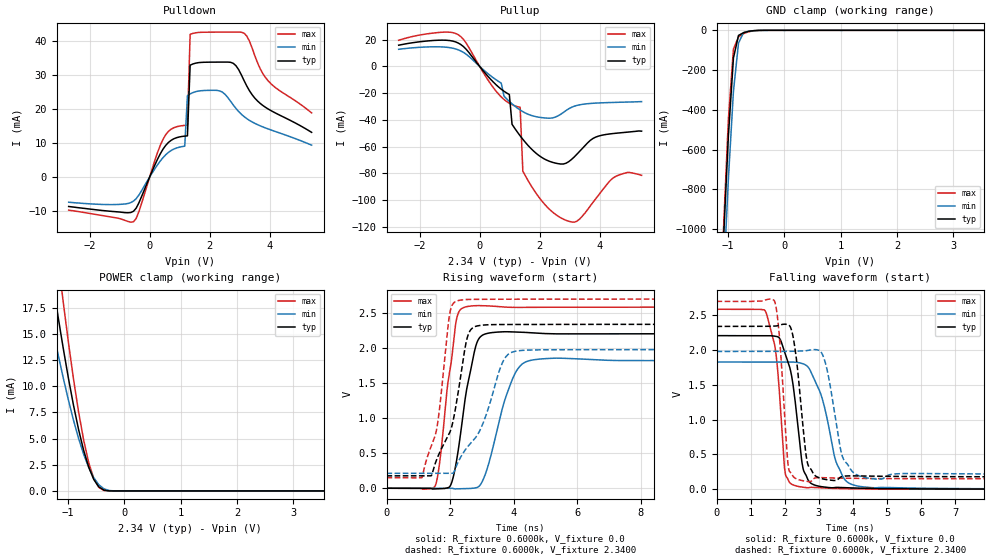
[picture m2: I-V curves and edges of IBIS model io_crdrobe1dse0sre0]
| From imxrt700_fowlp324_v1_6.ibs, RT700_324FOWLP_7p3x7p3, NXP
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[Model] io_crdrobe1dse0sre0
|   Model io_crdrobe1dse0sre0
| This model was characterised for following simulation conditions:
| External (pad) voltage:
|   - Typ: 2.34V,   - Min: 1.98V,   - Max: 2.7V
| Library cells for typ/min/max conditions are connected as defined below:
|  PAD_IO - External Pad
|  ipp_do - Core Input
|  ipp_obe - Output Buffer Enable
|  ASRCN3V3[3] - NC
|  ASRCN3V3[4] - NC
|  ASRCP3V3[4] - NC
|  REFAPBIAS3V3 - gnde
|  REFBAMPL3V3 - vdd1v8
|  REFCAMPH3V3 - vdd1v8
|  REFDNBIAS3V3 - vdd1v8
|  REFH3V3 - REFH3V3
|  REFL3V3 - REFL3V3
|  gnde - gnde
|  ipp_dse - gnde
|  ipp_ina235_3v - NC
|  ipp_ina40_3v - NC
|  ipp_ina_mux - NC
|  ipp_ind - NC
|  ipp_ind_1p8v - NC
|  ipp_ind_3v - NC
|  ipp_sre - gnde
|  vdd - vdd
|  vdd1v8 - vdd1v8
|  vdda - vdde3v3
|  vdde3v3 - vdde3v3
| All other pins connected to ground
Model_type I/O
Polarity   Non-Inverting
Enable   Active-High
Vinl =   0.7020V
Vinh =   1.6300V
Vmeas =  1.1700V
Cref =   15.0000pF
Rref =   0.6000k
Vref =   0.0V
C_comp   3.9951pF   3.8194pF   4.1033pF
|C_comp_pullup   0.5141pF   0.5880pF   0.4995pF
|C_comp_pulldown   2.0718pF   2.1610pF   1.8544pF
[Model Spec]
| variable   typ   min   max
Vinh   1.6300V   NA   NA
Vinl   0.7020V   NA   NA
Vref   0.0V   0.0V   0.0V
Cref   15.0000pF   15.0000pF   15.0000pF
Rref   0.6000k   0.6000k   0.6000k
[Receiver Thresholds]
Vcross_high  =   0.0V
Vcross_low  =   0.0V
Vdiff_ac  =   0.0V
Vdiff_dc  =   0.0V
Tdiffslew_ac  =   0.0S
[Temperature Range]   25.0000   0.1250k   -40.0000
[Voltage Range]   2.3400V   1.9800V   2.7000V
[Pullup Reference]   2.3400V   1.9800V   2.7000V
[Pulldown Reference]   0.0V   0.0V   0.0V
[POWER Clamp Reference]   2.3400V   1.9800V   2.7000V
[GND Clamp Reference]   0.0V   0.0V   0.0V
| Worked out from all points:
|   slope of the pulldown table from 0 to 0.351 V, typ, clamps not added: 51.9 ohm
|   slope of the pullup table from 0 to 0.351 V, typ, clamps not added: 37.8 ohm
|   GND clamp passes 1 mA (typ) near -0.49 V on its own axis
|   POWER clamp passes 1 mA (typ) near -0.53 V on its own axis
|   rising waveform, R_fixture 0.6000k, V_fixture 0.0: 20-80 % time 460ps typ, 657ps min, 391ps max; typ from 0 V to 2.21 V
|   rising waveform, R_fixture 0.6000k, V_fixture 2.3400: 20-80 % time 658ps typ, 1.01ns min, 453ps max; typ from 0.177 V to 2.34 V
|   falling waveform, R_fixture 0.6000k, V_fixture 0.0: 20-80 % time 352ps typ, 552ps min, 257ps max; typ from 2.21 V to 0 V
|   falling waveform, R_fixture 0.6000k, V_fixture 2.3400: 20-80 % time 263ps typ, 360ps min, 204ps max; typ from 2.34 V to 0.177 V
[Pulldown]
|Voltage   I(typ)   I(min)   I(max)
-2.7V     -8.67mA    -7.41mA    -9.74mA
-450mV    -9.161mA   -6.365mA   -12.21mA
450mV     8.254mA    5.751mA    11.17mA
1.17V     12.03mA    9.072mA    15.18mA
1.26V     12.11mA    23.94mA    15.24mA
1.35V     32.9mA     24.45mA    41.96mA
2.34V     33.8mA     25.32mA    42.61mA
2.79V     33.43mA    21.16mA    42.62mA
3.15V     28.33mA    17.76mA    42.29mA
3.51V     23.17mA    15.76mA    35.6mA
3.96V     19.96mA    14.11mA    28.19mA
5.4V      13.14mA    9.377mA    18.85mA
[Pullup]
|Voltage   I(typ)   I(min)   I(max)
-2.7V     15.88mA    12.82mA    19.56mA
-540mV    14.85mA    10.51mA    20.28mA
720mV     -17.09mA   -12.5mA    -22.86mA
990mV     -21.04mA   -26.21mA   -27.62mA
1.08V     -43.37mA   -28.03mA   -28.69mA
1.35V     -52.01mA   -32.66mA   -30.61mA
1.44V     -54.61mA   -33.9mA    -78.45mA
2.7V      -73.13mA   -35.9mA    -113.4mA
3.24V     -65.84mA   -29.25mA   -116mA
3.87V     -52.96mA   -27.49mA   -99.18mA
4.5V      -50.17mA   -26.97mA   -82.85mA
5.4V      -48.51mA   -26.37mA   -81.57mA
[GND_clamp]
|Voltage   I(typ)   I(min)   I(max)
-2.7V     -12.91A    -12.88A    -13.56A
-1.08V    -1.077A    -1.286A    -1.025A
-990mV    -533.6mA   -749.4mA   -449.1mA
-900mV    -139.2mA   -307mA     -94.25mA
-810mV    -25.49mA   -63.91mA   -32.87mA
-720mV    -11.78mA   -11.41mA   -16.65mA
-540mV    -1.684mA   -1.901mA   -2.149mA
-360mV    -36.04uA   -133.3uA   -15.05uA
5.4V      0A         0A         0A
[POWER_clamp]
|Voltage   I(typ)   I(min)   I(max)
-2.7V     73.96mA    57.58mA    95.4mA
-1.44V    26.15mA    20.18mA    34.67mA
-1.35V    22.86mA    17.7mA     30.34mA
-1.26V    19.66mA    15.3mA     26.09mA
-1.17V    16.56mA    12.98mA    21.97mA
-1.08V    13.59mA    10.78mA    17.99mA
-900mV    8.212mA    6.776mA    10.73mA
-720mV    3.9mA      3.518mA    4.888mA
-630mV    2.284mA    2.252mA    2.724mA
-540mV    1.103mA    1.268mA    1.195mA
-360mV    77.93uA    204.3uA    41.52uA
5.4V      0A         0A         0A
[Ramp]
| variable   typ   min   max
dV/dt_r  1.3244/0.4605n   1.0971/0.6570n   1.5519/0.3913n
dV/dt_f  1.2978/0.2633n   1.0605/0.3600n   1.5299/0.2036n
R_load = 0.6000k
[Rising Waveform]
R_fixture= 0.6000k
V_fixture= 0.0
V_fixture_min= 0.0
V_fixture_max= 0.0
|time   V(typ)   V(min)   V(max)
0s        133.2nV    3.451uV    44.06nV
1.533ns   -9.527mV   -1.01mV    33.33mV
1.687ns   -8.499mV   -1.147mV   416.8mV
1.988ns   22.09mV    -664.7uV   1.664V
2.2ns     382mV      -8.58mV    2.404V
2.686ns   1.772V     -1.261mV   2.602V
3.091ns   2.199V     176.5mV    2.604V
4.056ns   2.231V     1.647V     2.581V
4.932ns   2.208V     1.848V     2.583V
60ns      2.207V     1.829V     2.586V
[Rising Waveform]
R_fixture= 0.6000k
V_fixture= 2.3400
V_fixture_min= 1.9800
V_fixture_max= 2.7000
|time   V(typ)   V(min)   V(max)
0s        177mV      212.5mV    150.2mV
1.122ns   176.2mV    212.4mV    156.7mV
1.417ns   183.5mV    212mV      613.7mV
1.589ns   421.2mV    211.6mV    868.7mV
2.007ns   813.8mV    212.9mV    2.532V
2.406ns   1.817V     498.7mV    2.689V
2.745ns   2.299V     691mV      2.696V
3.709ns   2.337V     1.845V     2.698V
4.318ns   2.337V     1.969V     2.699V
60ns      2.34V      1.98V      2.7V
[Falling Waveform]
R_fixture= 0.6000k
V_fixture= 0.0
V_fixture_min= 0.0
V_fixture_max= 0.0
|time   V(typ)   V(min)   V(max)
0s        2.207V     1.828V     2.586V
1.423ns   2.208V     1.828V     2.567V
1.71ns    2.2V       1.828V     2.059V
1.854ns   2.165V     1.827V     1.328V
2.026ns   1.93V      1.829V     204.5mV
2.661ns   157.3mV    1.769V     19.67mV
3.078ns   35.66mV    1.338V     18.06mV
3.695ns   23.16mV    190.9mV    7.396mV
4.556ns   10.58mV    21.93mV    2.643mV
60ns      2.996uV    16.17uV    1.711uV
[Falling Waveform]
R_fixture= 0.6000k
V_fixture= 2.3400
V_fixture_min= 1.9800
V_fixture_max= 2.7000
|time   V(typ)   V(min)   V(max)
0s        2.34V      1.98V      2.7V
1.696ns   2.344V     1.98V      2.709V
1.838ns   2.359V     1.979V     2.232V
2.109ns   2.361V     1.981V     313.5mV
2.316ns   1.977V     1.984V     155.7mV
2.693ns   337.7mV    1.997V     109.5mV
3.151ns   143.5mV    1.884V     164.7mV
3.73ns    185.8mV    425.8mV    157.1mV
4.681ns   186.1mV    145.3mV    152.4mV
60ns      177mV      212.6mV    150.2mV
